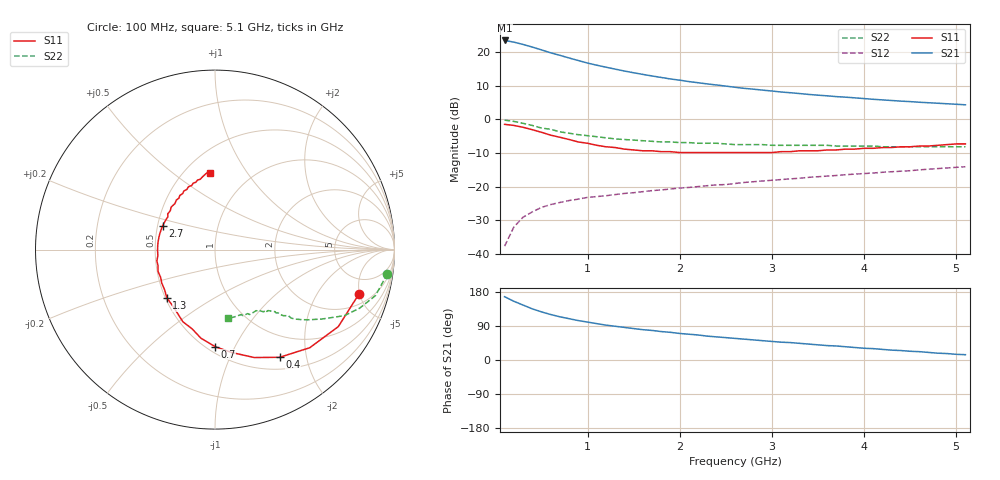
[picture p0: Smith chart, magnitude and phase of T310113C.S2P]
!AT-31011
!S and NOISE PARAMETERS at Vce=2.7V  Ic=5mA.  LAST UPDATED 03-06-95
# ghz s ma r 50
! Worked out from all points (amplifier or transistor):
!   51 points, 100 MHz to 5.1 GHz, reference 50 ohm
!   highest |S21| = 23.4 dB at 100 MHz (marker M1)
!   |S21| within 3 dB of that: start of sweep to 522.5 MHz
!   unconditionally stable (mu >= 1): 1.836 GHz to end of sweep
!   at 900 MHz: K = 0.64, MSG = 20.6 dB, |S12| = -23.7 dB
!   at 2.6 GHz: K = 1.15, MAG = 12.0 dB, |S12| = -19.1 dB
!   at 5.1 GHz: K = 1.09, MAG = 7.3 dB, |S12| = -14.1 dB
!   lowest NFmin = 0.70 dB at 100 MHz
!   S11 on the Smith chart (normalised r, x): 100 MHz: 2.97, -4.96; 400 MHz: 0.66, -1.56; 700 MHz: 0.55, -0.84; 1.3 GHz: 0.51, -0.32; 2.7 GHz: 0.53, +0.15; 5.1 GHz: 0.65, +0.69
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0.1  0.84 -17.0  14.83 167.0  0.013 81.0  0.97 -8.0
0.2  0.81 -32.0  14.01 155.0  0.025 73.0  0.93 -16.0
0.3  0.76 -46.0  12.94 145.0  0.035 66.0  0.87 -22.0
0.4  0.7 -59.0  11.84 135.0  0.042 61.0  0.81 -27.0
0.5  0.64 -70.0  10.74 127.0  0.049 56.0  0.74 -31.0
0.6  0.58 -81.0  9.71 120.0  0.054 53.0  0.71 -33.0
0.7  0.54 -90.0  8.92 114.0  0.058 51.0  0.65 -37.0
0.8  0.5 -99.0  8.14 109.0  0.062 49.0  0.62 -39.0
0.9  0.46 -106.0  7.46 104.0  0.065 48.0  0.59 -41.0
1  0.44 -114.0  6.84 100.0  0.069 47.0  0.57 -42.0
1.2  0.39 -128.0  5.94 92.0  0.073 46.0  0.53 -44.0
1.3  0.38 -135.0  5.56 89.0  0.076 45.0  0.51 -45.0
1.6  0.34 -153.0  4.64 80.0  0.084 45.0  0.48 -46.0
1.8  0.33 -164.0  4.18 75.0  0.089 45.0  0.46 -48.0
2.1  0.32 -179.0  3.63 68.0  0.097 45.0  0.45 -50.0
2.3  0.32 172.0  3.35 63.0  0.103 45.0  0.44 -51.0
2.6  0.32 160.0  2.99 57.0  0.111 45.0  0.42 -54.0
2.7  0.32 156.0  2.88 55.0  0.115 45.0  0.42 -54.0
3.1  0.33 143.0  2.54 47.0  0.127 44.0  0.41 -57.0
3.5  0.34 131.0  2.28 40.0  0.14 43.0  0.41 -61.0
4.3  0.38 110.0  1.9 26.0  0.166 40.0  0.39 -69.0
5.1  0.43 94.0  1.64 14.0  0.197 36.0  0.39 -79.0
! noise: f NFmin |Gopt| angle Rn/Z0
0.1  0.7  0.83  5  0.86
0.5  0.8  0.76  13  0.75
0.9  0.9  0.69  30  0.64
1.8  1.3  0.54  72  0.4
2.4  1.7  0.43  106  0.25
